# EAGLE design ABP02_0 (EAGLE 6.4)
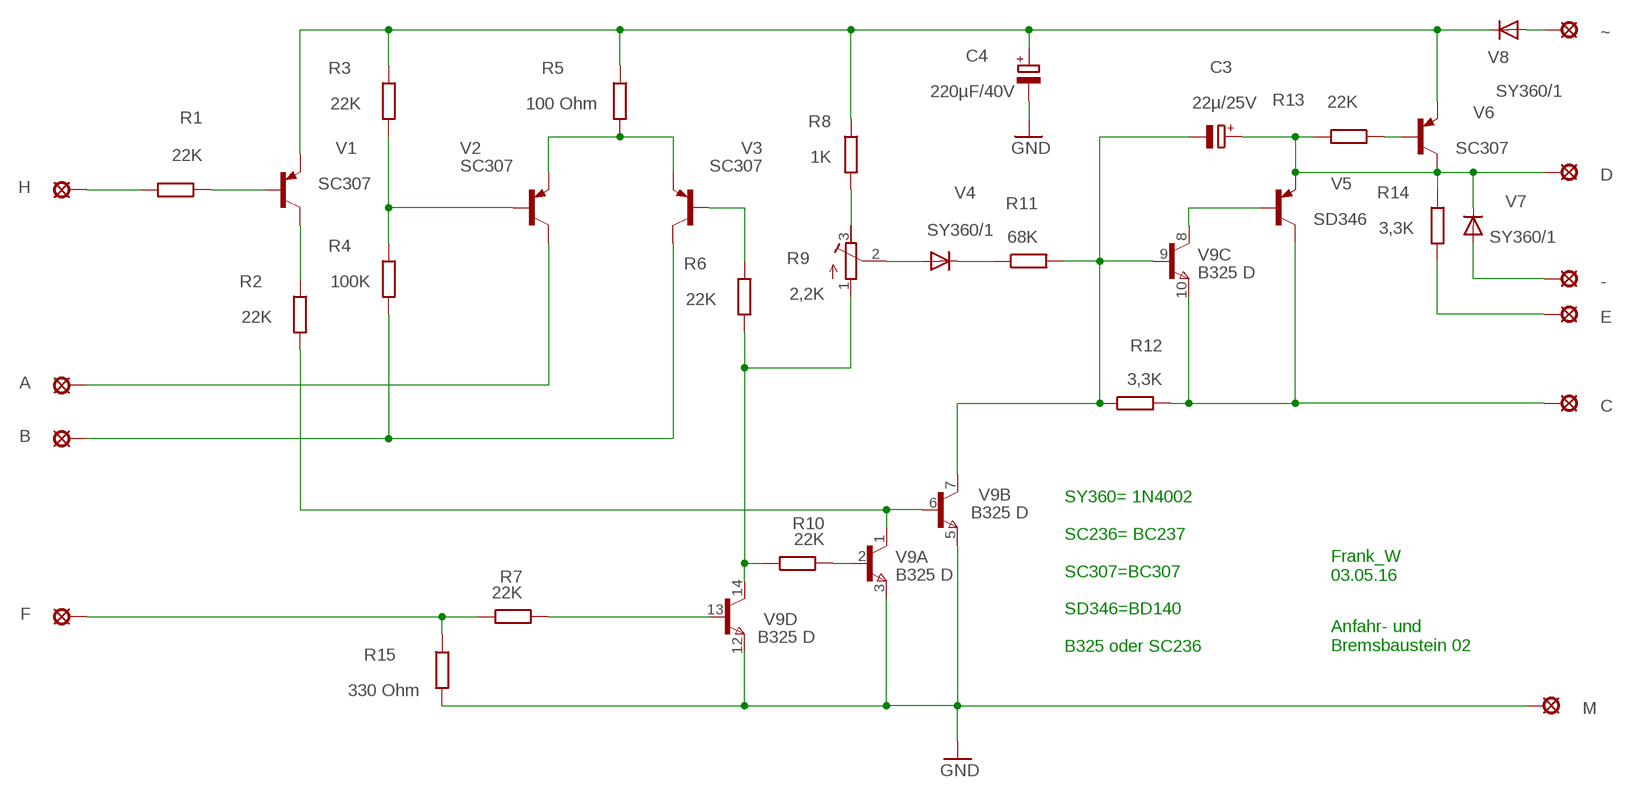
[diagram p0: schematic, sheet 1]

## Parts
-  LSP10  [LSP10]
A  LSP10  [LSP10]
B  LSP10  [LSP10]
C  LSP10  [LSP10]
C3  22µ/25V  CPOL-EUE5-5  [E5-5]
C4  220µF/40V  CPOL-EUE30-10AXIAL  [E30-10]
D  LSP10  [LSP10]
E  LSP10  [LSP10]
F  LSP10  [LSP10]
H  LSP10  [LSP10]
M  LSP10  [LSP10]
R1  22K  R-EU_0207/12  [0207/12]
R2  22K  R-EU_0207/12  [0207/12]
R3  22K  R-EU_0207/12  [0207/12]
R4  100K  R-EU_0207/12  [0207/12]
R5  100 Ohm  R-EU_0207/12  [0207/12]
R6  22K  R-EU_0207/12  [0207/12]
R7  22K  R-EU_0207/12  [0207/12]
R8  1K  R-EU_0207/12  [0207/12]
R9  2,2K  R-TRIMM64P  [RTRIM64P]
R10  22K  R-EU_0207/12  [0207/12]
R11  68K  R-EU_0207/12  [0207/12]
R12  3,3K  R-EU_0207/12  [0207/12]
R13  22K  R-EU_0207/12  [0207/12]
R14  3,3K  R-EU_0207/12  [0207/12]
R15  330 Ohm  R-EU_0207/12  [0207/12]
V1  SC307  BC327  [TO92]
V2  SC307  BC327  [TO92]
V3  SC307  BC327  [TO92]
V4  SY360/1  1N4004  [DO41-10]
V5  SD346  BD140  [TO126]
V6  SC307  BC327  [TO92]
V7  SY360/1  1N4004  [DO41-10]
V8  SY360/1  1N4004  [DO41-10]
V9  B325 D  MAT-04Y  [DIL14]
~  LSP10  [LSP10]

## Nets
GND: C4.- M.MP R15.2 V9.3(A:E) V9.5(B:E) V9.12(D:E)
N$1: C3.+ D.MP R13.2 R14.1 V5.1(E) V6.3(C) V7.C
N$2: H.MP R1.2
N$3: R1.1 V1.2(B)
N$4: R3.2 R4.1 V2.2(B)
N$5: R2.1 V1.3(C)
N$6: R5.2 V2.1(E) V3.1(E)
N$7: C4.+ R3.1 R5.1 R8.1 V1.1(E) V6.1(E) V8.C
N$8: A.MP V2.3(C)
N$9: R13.1 V6.2(B)
N$10: B.MP R4.2 V3.3(C)
N$11: R9.2(S) V4.A
N$12: R8.2 R9.3(E)
N$13: R6.2 R9.1(A) R10.1 V9.14(D:C)
N$14: R6.1 V3.2(B)
N$15: R11.1 V4.C
N$16: F.MP R7.1 R15.1
N$17: R7.2 V9.13(D:B)
N$18: E.MP R14.2
N$19: R10.2 V9.2(A:B)
N$20: R2.2 V9.1(A:C) V9.6(B:B)
N$21: C3.- R11.2 R12.1 V9.7(B:C) V9.9(C:B)
N$22: V5.3(B) V9.8(C:C)
N$23: C.MP R12.2 V5.2(C) V9.10(C:E)
N$24: -.MP V7.A
N$25: V8.A ~.MP

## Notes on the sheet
- Frank_W
  03.05.16
- SY360= 1N4002
  
  SC236= BC237
  
  SC307=BC307
  
  SD346=BD140
  
  B325 oder SC236
- Anfahr- und
  Bremsbaustein 02

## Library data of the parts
- A B C D E F H M ~ = solpad:LSP10: SOLDER PAD
C3 C4 = rcl:CPOL-EU: POLARIZED CAPACITOR, European symbol
R1-R8 R10-R15 = rcl:R-EU_: RESISTOR, European symbol
R9 = rcl:R-TRIMM: Trimm resistor
V1-V3 V6 = transistor-pnp:BC327: PNP Transistor
V4 V7 V8 = diode:1N4004: DIODE
V5 = transistor-pnp:BD140: PNP Transistor
V9 = linear:MAT-04: Quad TRANSISTOR

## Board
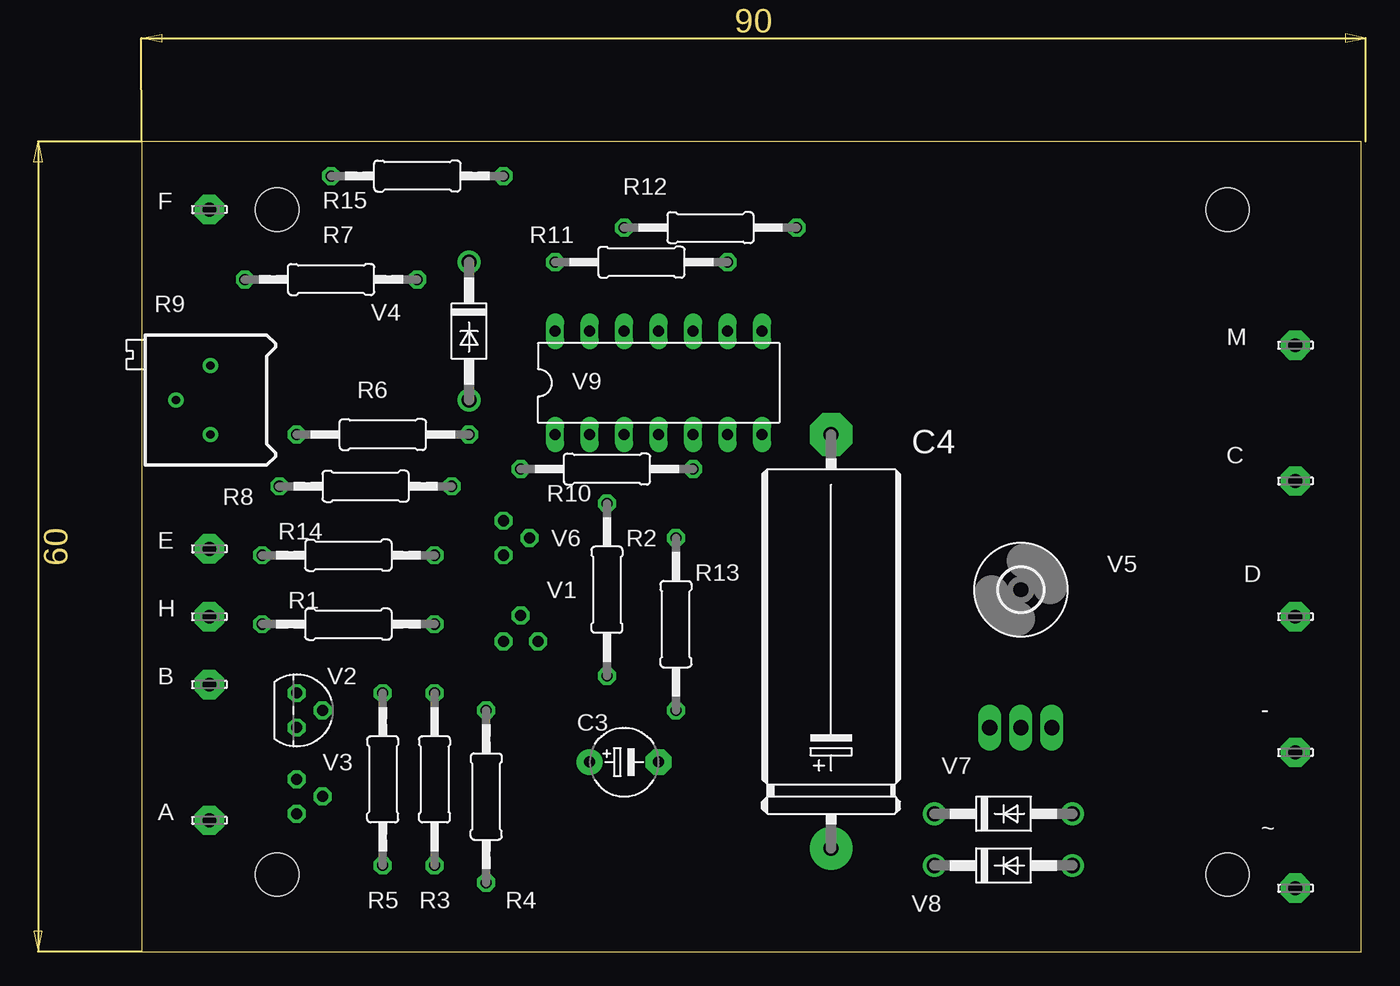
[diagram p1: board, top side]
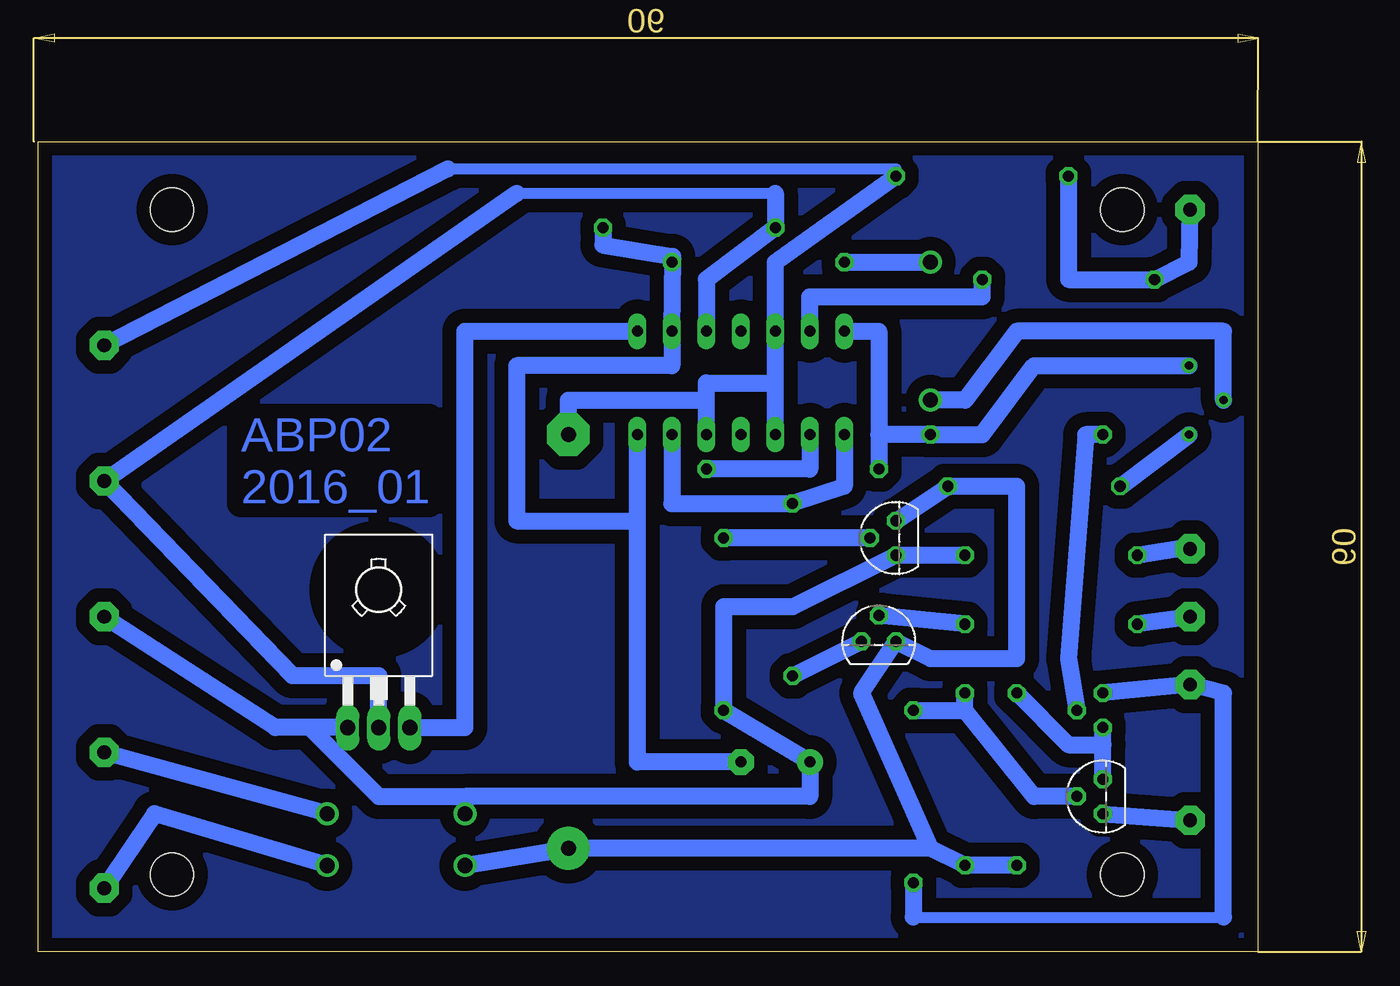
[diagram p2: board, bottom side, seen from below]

Size 98.09 x 67.61 mm. Coordinates in mm from the lower left corner, seen from the top.
Outline: 7.92,0 97.76,0 97.76,59.68 7.92,59.68 7.92,0
Copper layers (1*16): Top 0.035mm / dielectric 1.5mm / Bottom 0.035mm
Design rules "default *": minimum track width 20mil, minimum drill 24mil, track to track 8mil, track to pad 8mil, pad to pad 8mil, via to via 8mil, smd to smd 8mil, copper to edge 40mil, drill to drill 8mil, minimum pad ring 10mil, minimum via ring 8mil, stop-mask expansion 4mil, vias tented up to drill 0mil, thermal gap 20mil
Holes 3.2 mm at 87.92,54.68 87.92,5.68 17.92,5.68 17.92,54.68

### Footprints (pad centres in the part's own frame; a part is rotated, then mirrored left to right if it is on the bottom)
LSP10 = drill 1.016 pad 2.159 octagon: MP 0,0
E5-5 = drill 0.813 pad 1.905: + -2.54,0 | drill 0.813 pad 1.905 octagon: - 2.54,0
E30-10 = drill 1.118 pad 3.15: + -15.24,0 | drill 1.118 pad 3.15 octagon: - 15.24,0
0207/12 = drill 0.813 octagon: 1 -6.35,0; 2 6.35,0
RTRIM64P = drill 0.61: 1 0,-2.54; 2 2.54,0; 3 0,2.54
3,2 = hole 3.2: 0,0
TO92 = drill 0.813 octagon: 1 1.27,0; 2 0,1.905; 3 -1.27,0
DO41-10 = drill 1.118: A 5.08,0; C -5.08,0
TO126 = drill 1.118 long: 1 -2.286,-5.08; 2 0,-5.08; 3 2.286,-5.08 | hole 3.302: 0,5.08
DIL14 = drill 0.813 long: 1 -7.62,-3.81; 2 -5.08,-3.81; 3 -2.54,-3.81; 4 0,-3.81; 5 2.54,-3.81; 6 5.08,-3.81; 7 7.62,-3.81; 8 7.62,3.81; 9 5.08,3.81; 10 2.54,3.81; 11 0,3.81; 12 -2.54,3.81; 13 -5.08,3.81; 14 -7.62,3.81

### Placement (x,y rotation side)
-  92.92,14.68 0 top
A  12.92,9.68 0 top
B  12.92,19.68 0 top
C  92.92,34.68 0 top
C3  43.48,13.97 0 top
C4  58.72,22.86 90 top
D  92.92,24.68 0 top
E  12.92,29.68 0 top
F  12.92,54.68 0 top
H  12.92,24.68 0 top
M  92.92,44.68 0 top
R1  23.16,24.13 180 top
R2  42.21,26.67 90 top
R3  29.51,12.7 90 top
R4  33.32,11.43 270 top
R5  25.7,12.7 90 top
R6  25.7,38.1 0 top
R7  21.89,49.53 0 top
R8  24.43,34.29 180 top
R9  13,40.64 180 top
R10  42.21,35.56 0 top
R11  44.75,50.8 0 top
R12  49.83,53.34 180 top
R13  47.29,24.13 270 top
R14  23.16,29.21 180 top
R15  28.24,57.15 0 top
U$1  [3,2]  72.69,26.67 0 top
V1  35.86,22.86 0 bottom
V2  19.35,11.43 90 bottom
V3  19.35,17.78 270 top
V4  32.05,45.72 270 top
V5  72.69,21.59 0 bottom
V6  34.59,30.48 90 bottom
V7  71.42,10.16 0 top
V8  71.42,6.35 0 top
V9  46.02,41.91 0 top
~  92.92,4.68 0 top

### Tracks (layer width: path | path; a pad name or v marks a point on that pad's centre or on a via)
GND
  Bottom 0.813: 67.61,57.68 34.59,57.68 R15.2
  Bottom 1.27: V9.3 43.48,41.91 | 43.48,41.91 V9.12 43.48,50.8 R15.2 | 43.48,41.91 48.56,41.91 48.56,40.64 | M.MP 67.61,57.68 | V9.5 48.56,40.64 | C4.- 58.72,40.64 48.56,40.64
N$1
  Bottom 1.27: 66.34,11.43 40.94,11.43 C3.+ R13.2 47.29,25.4 42.21,25.4 V6.3 R14.1 | V7.C 66.34,11.43 | 93.01,24.68 D.MP 80.31,16.51 77.77,16.51 | 66.34,11.43 72.69,11.43 77.77,16.51 | V5.1 77.77,16.51
N$2
  Bottom 1.27: H.MP R1.2
N$3
  Bottom 1.27: R1.1 V1.2
N$4
  Bottom 1.27: R4.1 29.51,17.78 | 29.51,17.78 R3.2 | V2.2 24.43,11.43 29.51,17.78
N$5
  Bottom 1.27: R2.1 V1.3
N$6
  Bottom 1.27: R5.2 21.89,15.24 19.35,15.24 | 19.35,15.24 V3.1 | V2.1 19.35,15.24
N$7
  Bottom 1.27: V8.C C4.+ 32.05,7.62 | R5.1 R3.1 32.05,7.62 | V6.1 R8.1 25.7,34.29 25.7,21.59 32.05,21.59 V1.1 37.13,19.05 32.05,7.62
N$8
  Bottom 1.27: V2.3 A.MP
N$9
  Bottom 1.27: V6.2 R13.1
N$10
  Bottom 0.813: 33.32,2.54 10.46,2.54
  Bottom 1.27: V3.3 B.MP 10.46,19.05 10.46,2.54 | R4.2 33.32,2.54
N$11
  Bottom 1.27: R9.2 10.46,45.72 25.7,45.72 29.51,40.64 V4.A
N$12
  Bottom 1.27: R8.2 R9.3
N$13
  Bottom 1.27: 35.86,38.1 R6.2 28.24,38.1 24.43,43.18 R9.1 | 35.86,38.1 R10.1 | V9.14 35.86,45.72 35.86,38.1
N$14
  Bottom 1.27: R6.1 20.62,38.1 21.89,21.59 V3.2
N$15
  Bottom 1.27: R11.1 V4.C
N$16
  Bottom 1.27: F.MP 13,50.8 R7.1 21.89,49.53 R15.1
N$17
  Bottom 1.27: V9.13 40.94,48.26 28.24,48.26 R7.2
N$18
  Bottom 1.27: E.MP 13.8,29.68 R14.2
N$19
  Bottom 1.27: V9.2 40.94,35.56 R10.2
N$20
  Bottom 1.27: V9.6 51.1,33.02 R2.2 38.4,34.29 V9.1
N$21
  Bottom 1.27: R12.1 56.18,52.07 51.03,51.21 | 51.03,51.21 R11.2 | 51.03,51.21 V9.9 51.1,43.18 62.53,43.18 62.53,31.75 53.64,31.75 | 53.64,31.75 V9.7 | C3.- 53.64,13.97 53.64,31.75
N$22
  Bottom 1.27: V5.3 66.34,16.51 66.34,45.72 V9.8
N$23
  Bottom 0.813: 62.53,55.88 43.48,55.88
  Bottom 1.27: V9.10 48.56,49.53 R12.2 43.48,55.88 | 62.53,55.88 C.MP 79.04,20.32 72.69,20.32 V5.2
N$24
  Bottom 1.27: V7.A 76.41,10.16 -.MP
N$25
  Bottom 1.27: V8.A 89.2,10.16 ~.MP
N$26
  pour Bottom (isolate 1.016): 7.92,59.69 98.09,59.69 98.09,0 7.92,0

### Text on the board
Bottom: ABP02 / 2016_01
